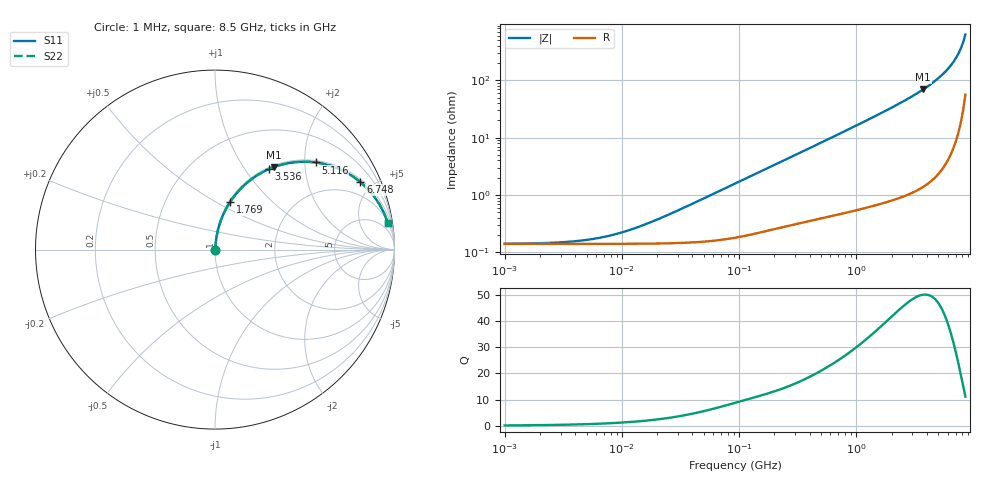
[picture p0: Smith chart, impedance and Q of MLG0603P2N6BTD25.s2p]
! S-Parameter Data Generated by TDK Corporation
! Copyright(C) 2025 TDK Corporation.
! All Rights Reserved.
! TDK P/N: MLG0603P2N6BTD25 (SMD / SMT Inductor (Coil))
! Property: L=2.6nH at 500MHz
! Size(LxWxT): 0.6x0.3x0.3mm
! Model Type: s2p (Touchstone File Format Version 1.0)
! Frequency: DC=Yes Start=1MHz Stop=8500MHz 198points Log-sweep
! Model Generated on Feb. 6, 2025
! Terms and conditions regarding TDK Simulation Models:
! 1)This simulation model is being provided solely for informational
!  purposes. Please refer to the specifications of the products in
!  terms of detailed characteristics of such products.
! 2)In no event shall TDK Corporation of any of its subsidiaries be
!  liable for any loss or damage arising, directly or indirectly,
!  from any information contained in this simulation model, including,
!  but not limited to loss or damages arising from any inaccuracies,
!  omissions or errors in connection with such information.
! 3)Any and all copyrights on this simulation model are owned by
!  TDK Corporation.  Duplication or redistribution of this simulation
!  model without prior written permission from TDK Corporation
!  is prohibited.
! 4)This simulation model is subject to any modification or change
!  without any prior notice.
! 5)Neither TDK Corporation nor any of its subsidiaries shall make any
!  warranty, express or implied, including but not limited to the
!  correctness, implied warranties of merchantability and fitness for
!  a particular purpose with respect to this simulation models.
! 6)The use of this simulation model shall be deemed to have consented
!  to the terms and conditions hereof.
! Port Assignments:
!  1 ---@@@--- 2
! Applicable Conditions:
!  Temperature = 25 degC
!  DC Bias Current = 0 A
!  Small Signal Operation
# Hz S MA R 50
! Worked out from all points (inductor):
!   197 points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, 1 MHz to 8.5 GHz, reference 50 ohm
!   read as one part in series: L = 2.74 nH near 25.31 MHz
!   highest Q = 50.1 at 3.703 GHz (marker M1), where L = 2.97 nH
!   S11 on the Smith chart (normalised r, x): 1 MHz: 1.00, +0.00; 1.769 GHz: 1.01, +0.59; 3.536 GHz: 1.03, +1.30; 5.116 GHz: 1.05, +2.27; 6.748 GHz: 1.13, +4.23; 8.5 GHz: 2, +13
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1000000  0.001409 7.0  0.9986 -0.0  0.9986 -0.0  0.001409 7.0
2517452  0.001464 17.2  0.9986 -0.0  0.9986 -0.0  0.001464 17.2
4587603  0.001607 29.4  0.9986 -0.0  0.9986 -0.0  0.001607 29.4
6636977  0.001807 39.1  0.9986 -0.1  0.9986 -0.1  0.001807 39.1
9601846  0.002168 49.6  0.9986 -0.1  0.9986 -0.1  0.002168 49.6
2.10461e7  0.003889 68.3  0.9986 -0.2  0.9986 -0.2  0.003889 68.3
9.219544e7  0.01578 82.6  0.9981 -0.9  0.9981 -0.9  0.01578 82.6
4.229561e8  0.06898 83.1  0.9941 -4.0  0.9941 -4.0  0.06898 83.1
9.270694e8  0.1484 79.5  0.9838 -8.5  0.9838 -8.5  0.1484 79.5
1.769233e9  0.279 72.4  0.9533 -16.2  0.9533 -16.2  0.279 72.4
1.940355e9  0.3051 70.8  0.9449 -17.8  0.9449 -17.8  0.3051 70.8
2.680511e9  0.4165 64.2  0.9003 -24.6  0.9003 -24.6  0.4165 64.2
3.535948e9  0.54 56.2  0.8309 -32.7  0.8309 -32.7  0.54 56.2
3.703002e9  0.5632 54.6  0.8152 -34.3  0.8152 -34.3  0.5632 54.6
4.453958e9  0.6626 47.4  0.7357 -41.5  0.7357 -41.5  0.6626 47.4
5.115526e9  0.7419 40.9  0.6546 -47.9  0.6546 -47.9  0.7419 40.9
5.87536e9  0.8211 33.4  0.5509 -55.2  0.5509 -55.2  0.8211 33.4
6.748056e9  0.8934 24.9  0.4218 -63.2  0.4218 -63.2  0.8934 24.9
7.400733e9  0.9335 18.8  0.3218 -68.9  0.3218 -68.9  0.9335 18.8
7.750377e9  0.95 15.5  0.2681 -71.6  0.2681 -71.6  0.95 15.5
8.116539e9  0.9636 12.2  0.2123 -74.1  0.2123 -74.1  0.9636 12.2
8.5e9  0.9742 8.9  0.1548 -76.0  0.1548 -76.0  0.9742 8.9
